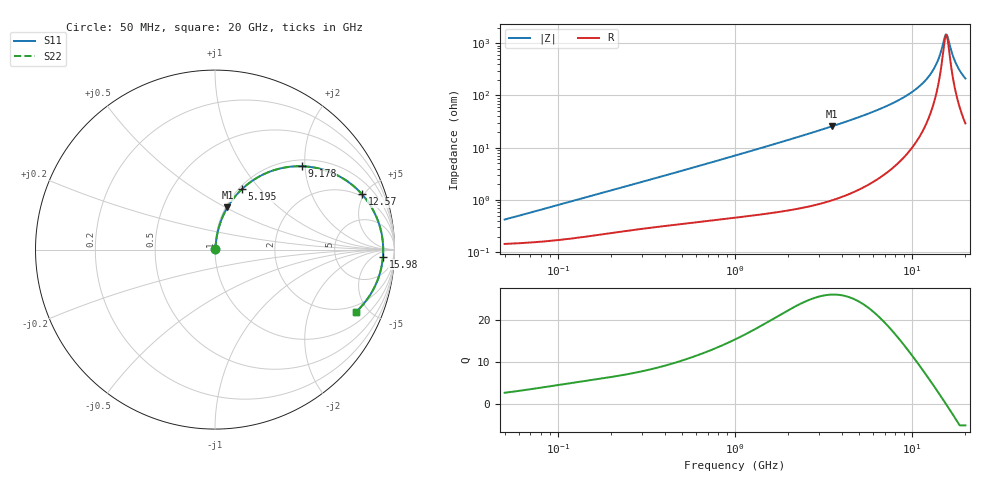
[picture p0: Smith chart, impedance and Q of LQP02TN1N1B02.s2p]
!Murata Part Number: LQP02TN1N1B02
!These Parameters are Measured in Series Mode Connection
!  o--[Z]--o
!Port1  Port2
!  o-------o
!Freq. Start=50[MHz] Stop=20[GHz], 401[Steps]
# Hz S RI R 50
!Freq.(Hz) S11(Real) S11(Imag) S21(Real) S21(Imag) S12(Real) S12(Imag) S22(Real) S22(Imag)
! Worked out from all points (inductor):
!   401 points, 50 MHz to 20 GHz, reference 50 ohm
!   read as one part in series: L = 1.26 nH near 55.53 MHz
!   highest Q = 26.1 at 3.519 GHz (marker M1), where L = 1.16 nH
!   self-resonance near 15.6 GHz
!   S11 on the Smith chart (normalised r, x): 50 MHz: 1.00, +0.01; 5.195 GHz: 1.03, +0.80; 9.178 GHz: 1.14, +1.93; 12.57 GHz: 1.83, +4.81; 15.98 GHz: 22, -14; 20 GHz: 1.58, -4.19
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5e7  0.00146 0.00396  0.9985 -0.00396  0.9985 -0.00396  0.00146 0.00396
1.364002e8  0.00205 0.0105  0.998 -0.0105  0.998 -0.0105  0.00205 0.0105
3.721004e8  0.0038 0.027  0.9962 -0.027  0.9962 -0.027  0.0038 0.027
1e9  0.00945 0.0696  0.9906 -0.0696  0.9906 -0.0696  0.00945 0.0696
2.728004e9  0.0433 0.1847  0.9567 -0.1847  0.9567 -0.1847  0.0433 0.1847
3.519108e9  0.0695 0.2358  0.9305 -0.2358  0.9305 -0.2358  0.0695 0.2358
5.194772e9  0.1497 0.3366  0.8503 -0.3366  0.8503 -0.3366  0.1497 0.3366
7.442007e9  0.315 0.4379  0.685 -0.4379  0.685 -0.4379  0.315 0.4379
9.178299e9  0.4837 0.4644  0.5163 -0.4644  0.5163 -0.4644  0.4837 0.4644
1.098561e10  0.6736 0.4181  0.3264 -0.4181  0.3264 -0.4181  0.6736 0.4181
1.257102e10  0.8182 0.3091  0.1818 -0.3091  0.1818 -0.3091  0.8182 0.3091
1.334722e10  0.8712 0.2369  0.1288 -0.2369  0.1288 -0.2369  0.8712 0.2369
1.396067e10  0.9025 0.1742  0.0975 -0.1742  0.0975 -0.1742  0.9025 0.1742
1.438523e10  0.9183 0.1292  0.0817 -0.1292  0.0817 -0.1292  0.9183 0.1292
1.527346e10  0.9357 0.0338  0.0643 -0.0338  0.0643 -0.0338  0.9357 0.0338
1.550395e10  0.937 0.00938  0.063 -0.00938  0.063 -0.00938  0.937 0.00938
1.573793e10  0.937 -0.0151  0.063 0.0151  0.063 0.0151  0.937 -0.0151
1.597544e10  0.9357 -0.0395  0.0643 0.0395  0.0643 0.0395  0.9357 -0.0395
1.696185e10  0.9179 -0.135  0.0821 0.135  0.0821 0.135  0.9179 -0.135
1.774144e10  0.8925 -0.2017  0.1075 0.2017  0.1075 0.2017  0.8925 -0.2017
1.88369e10  0.8452 -0.2807  0.1548 0.2807  0.1548 0.2807  0.8452 -0.2807
2e10  0.7868 -0.3457  0.2132 0.3457  0.2132 0.3457  0.7868 -0.3457
